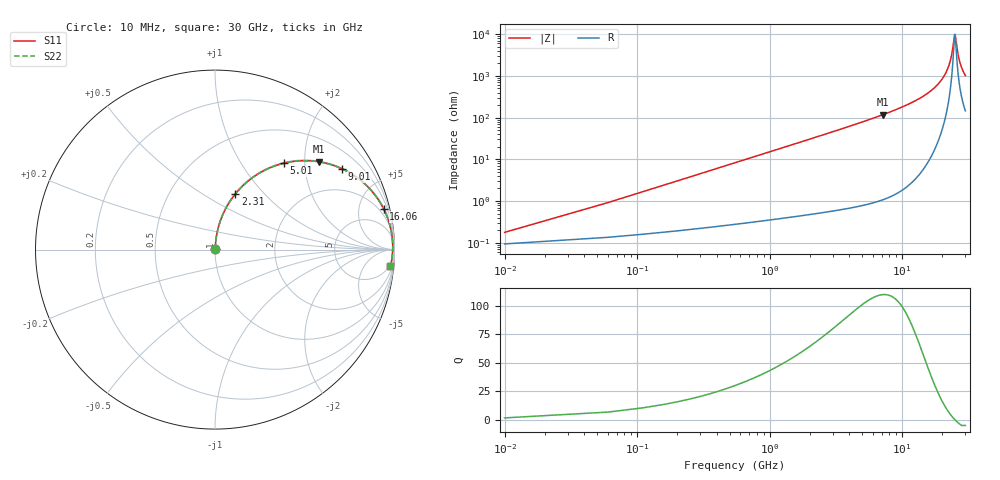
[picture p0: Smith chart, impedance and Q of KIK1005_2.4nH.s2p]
!version-3
!date-01.2023
!Series
# MHz S RI R 50
!Freq ReS11 ImS11 ReS21 ImS21 ReS12 ImS12 ReS22 ImS22
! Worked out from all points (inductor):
!   601 points, 10 MHz to 30 GHz, reference 50 ohm
!   read as one part in series: L = 2.4 nH near 160 MHz
!   highest Q = 110 at 7.16 GHz (marker M1), where L = 2.61 nH
!   self-resonance near 24.96 GHz
!   S11 on the Smith chart (normalised r, x): 10 MHz: 1.00, +0.00; 2.31 GHz: 1.01, +0.70; 5.01 GHz: 1.02, +1.57; 9.01 GHz: 1.03, +3.12; 16.06 GHz: 1.20, +8.24; 30 GHz: 4, -20
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10  0.000939 0.00151  0.9991 -0.00151  0.9991 -0.00151  0.000939 0.00151
210  0.00295 0.0315  0.9971 -0.0315  0.9971 -0.0315  0.00295 0.0315
260  0.00363 0.039  0.9964 -0.039  0.9964 -0.039  0.00363 0.039
560  0.00981 0.0834  0.9902 -0.0834  0.9902 -0.0834  0.00981 0.0834
1210  0.0358 0.1757  0.9642 -0.1757  0.9642 -0.1757  0.0358 0.1757
2310  0.1134 0.3099  0.8866 -0.3099  0.8866 -0.3099  0.1134 0.3099
5010  0.3837 0.4814  0.6163 -0.4814  0.6163 -0.4814  0.3837 0.4814
7160  0.5798 0.4891  0.4202 -0.4891  0.4202 -0.4891  0.5798 0.4891
9010  0.7074 0.4502  0.2926 -0.4502  0.2926 -0.4502  0.7074 0.4502
10010  0.7615 0.4212  0.2385 -0.4212  0.2385 -0.4212  0.7615 0.4212
15010  0.9218 0.259  0.0782 -0.259  0.0782 -0.259  0.9218 0.259
16060  0.9397 0.2265  0.0603 -0.2265  0.0603 -0.2265  0.9397 0.2265
20010  0.9791 0.1158  0.0209 -0.1158  0.0209 -0.1158  0.9791 0.1158
21710  0.9864 0.0735  0.0136 -0.0735  0.0136 -0.0735  0.9864 0.0735
22960  0.9892 0.0444  0.0108 -0.0444  0.0108 -0.0444  0.9892 0.0444
23760  0.99 0.0266  0.00997 -0.0266  0.00997 -0.0266  0.99 0.0266
24760  0.9901 0.00511  0.00992 -0.00511  0.00992 -0.00511  0.9901 0.00511
25010  0.9899 -0.000104  0.0101 0.000104  0.0101 0.000104  0.9899 -0.000104
26160  0.9886 -0.0234  0.0114 0.0234  0.0114 0.0234  0.9886 -0.0234
27010  0.9869 -0.0399  0.0131 0.0399  0.0131 0.0399  0.9869 -0.0399
28310  0.9834 -0.064  0.0166 0.064  0.0166 0.064  0.9834 -0.064
30000  0.9773 -0.0935  0.0227 0.0935  0.0227 0.0935  0.9773 -0.0935
